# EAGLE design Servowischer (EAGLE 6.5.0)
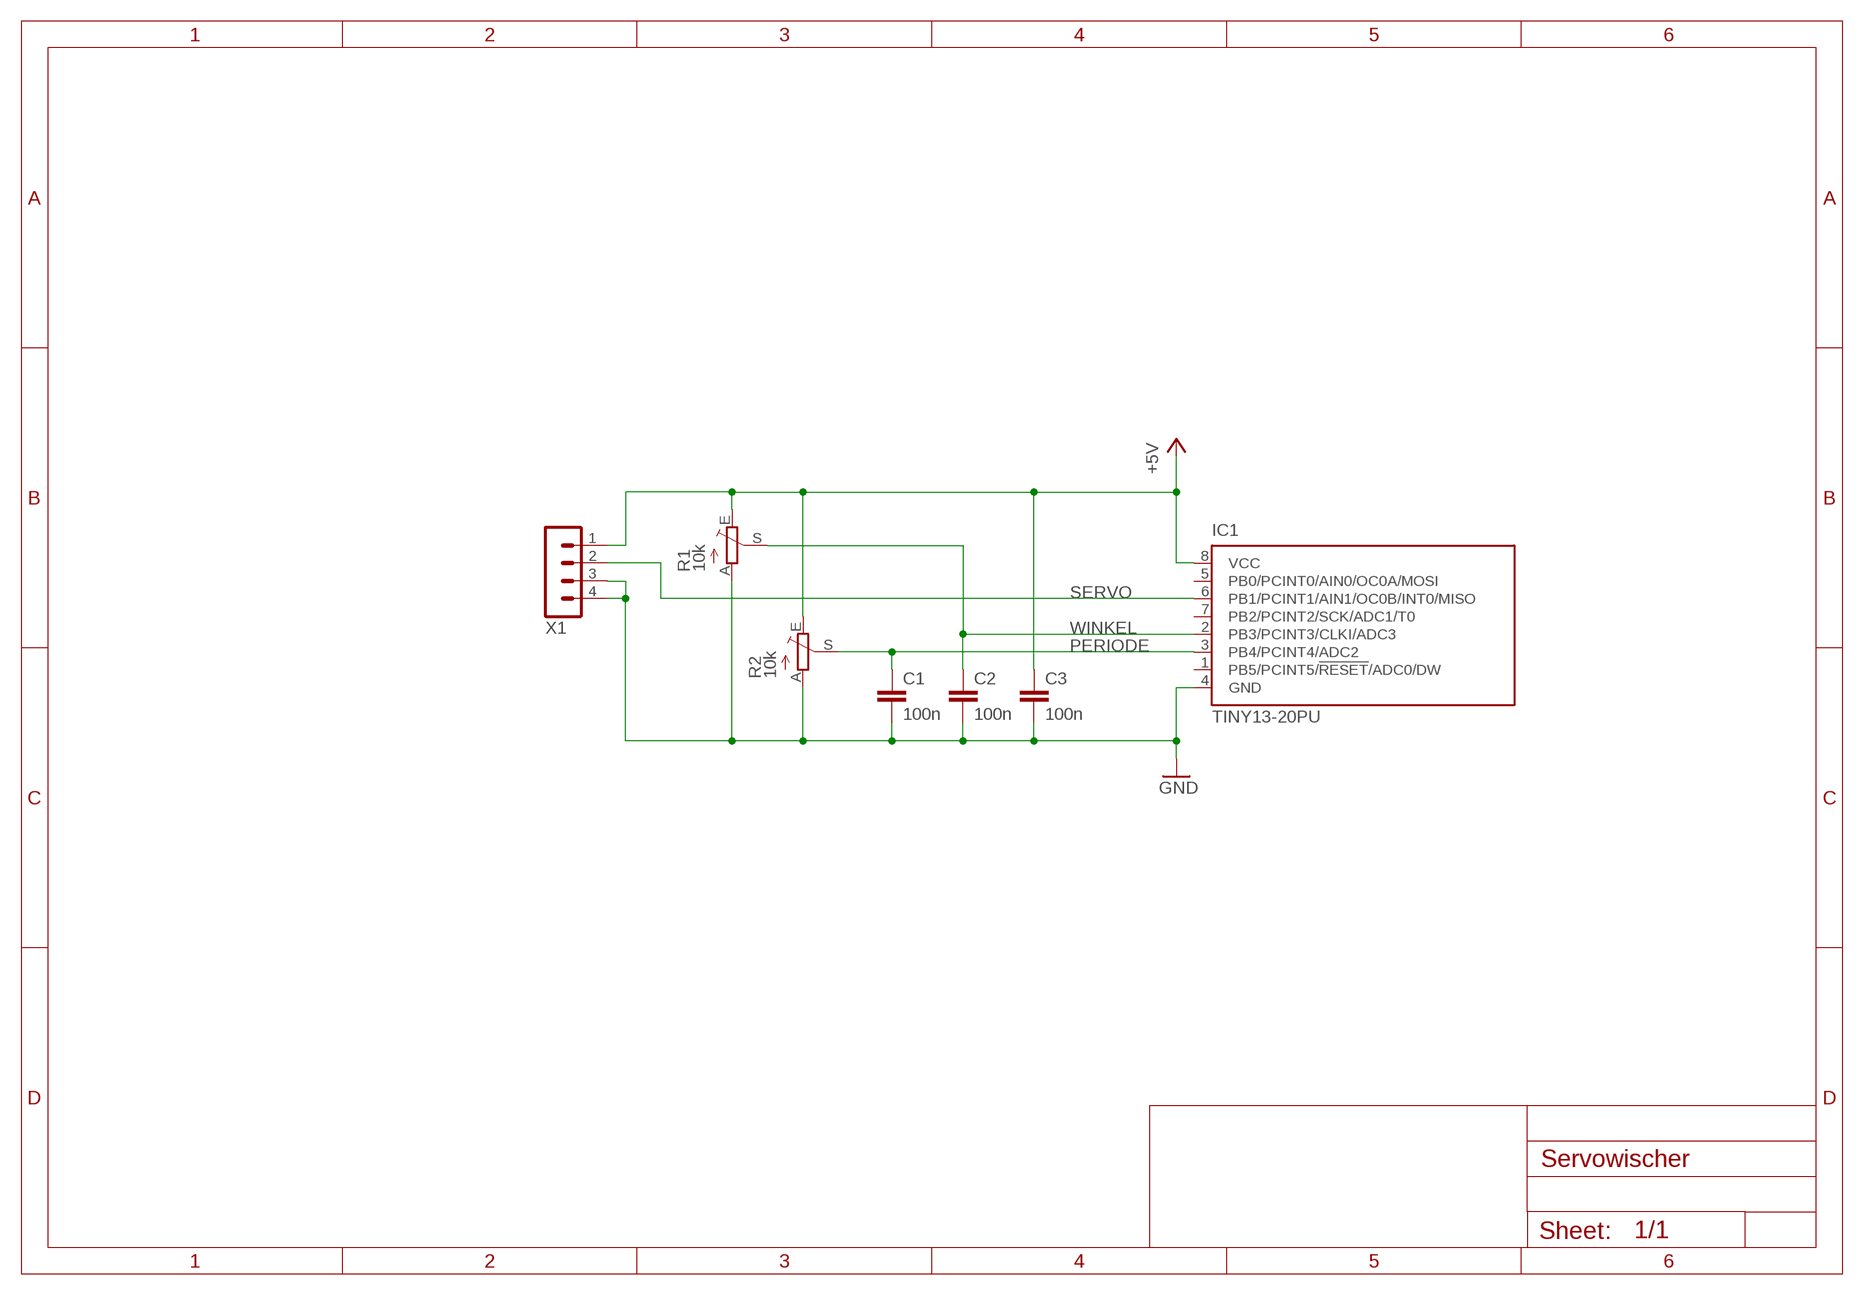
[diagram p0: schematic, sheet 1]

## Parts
C1  100n  C-EU050-024X044  [C050-024X044]
C2  100n  C-EU050-024X044  [C050-024X044]
C3  100n  C-EU050-024X044  [C050-024X044]
IC1  TINY13-20PU  [DIL08]
R1  10k  TRIM_EU-RJ9W  [RJ9W]
R2  10k  TRIM_EU-RJ9W  [RJ9W]
X1  MA04-1  [MA04-1]

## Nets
+5V: C3.1 IC1.8(VCC) R1.E R2.E X1.1
GND: C1.2 C2.2 C3.2 IC1.4(GND) R1.A R2.A X1.3 X1.4
PERIODE: C1.1 IC1.3(PB4/PCINT4/ADC2) R2.S
SERVO: IC1.6(PB1/PCINT1/AIN1/OC0B/INT0/MISO) X1.2
WINKEL: C2.1 IC1.2(PB3/PCINT3/CLKI/ADC3) R1.S
Unconnected: IC1.1(PB5/PCINT5/!RESET!/ADC0/DW) IC1.5(PB0/PCINT0/AIN0/OC0A/MOSI) IC1.7(PB2/PCINT2/SCK/ADC1/T0)

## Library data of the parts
C1-C3 = rcl:C-EU: CAPACITOR, European symbol
IC1 = atmel:TINY13: 8-bit AVR Microcontroller with 1K Bytes In-System Programmable Flash Source: http://www.atmel.com/dyn/resources/prod_documents/2535S.pdf; MPN: ATTINY13-20PU; OC_FARNELL: 9171550; OC_NEWARK: 96K6521
R1 R2 = pot:TRIM_EU-: POTENTIOMETER
X1 = con-lstb:MA04-1: PIN HEADER; OC_FARNELL: unknown; OC_NEWARK: unknown

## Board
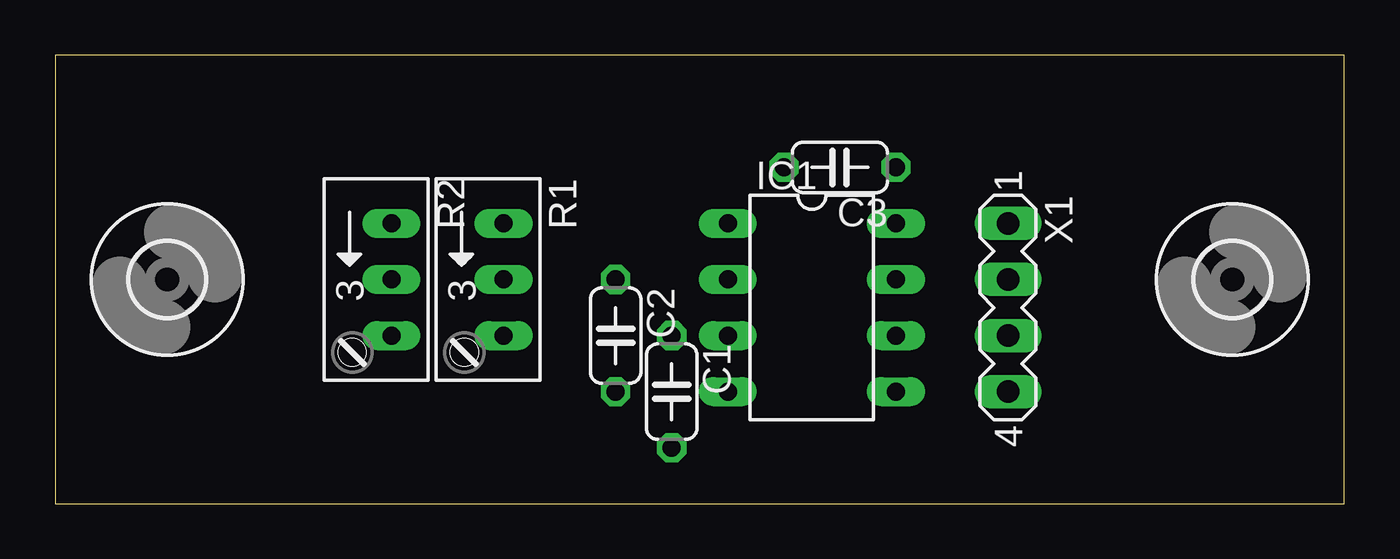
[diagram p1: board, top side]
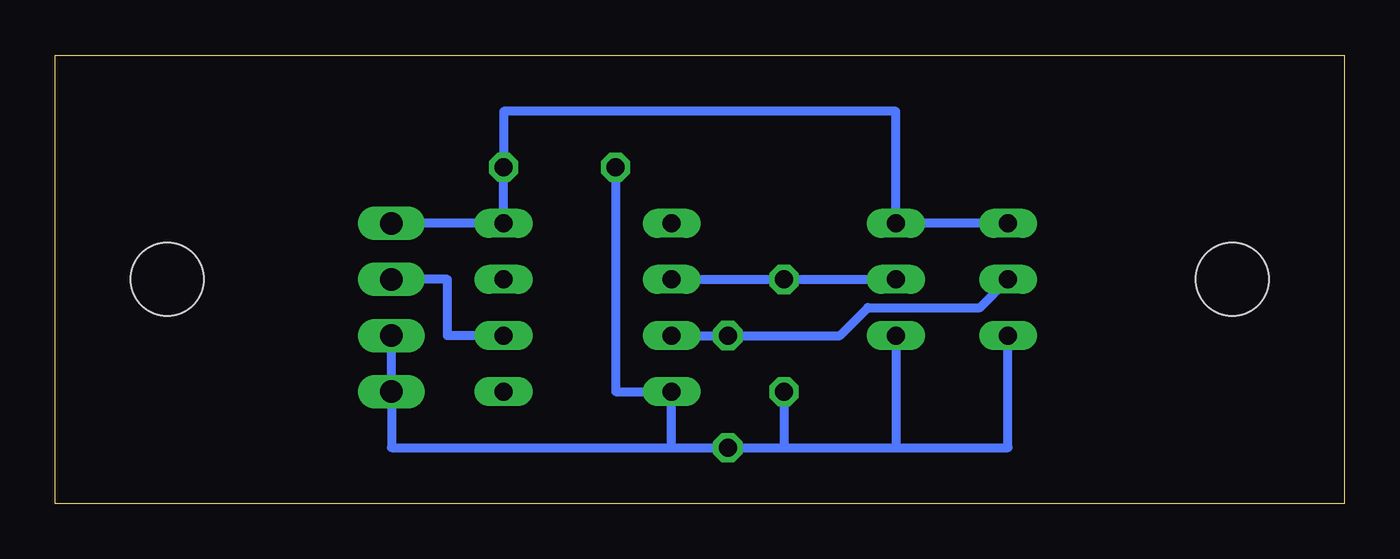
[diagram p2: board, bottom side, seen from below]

Size 58.42 x 20.32 mm. Coordinates in mm from the lower left corner, seen from the top.
Outline: 0,0 58.42,0 58.42,20.32 0,20.32 0,0
Copper layers (1*16): Top 0.035mm / dielectric 1.5mm / Bottom 0.035mm
Design rules "default": minimum track width 10mil, minimum drill 24mil, track to track 8mil, track to pad 8mil, pad to pad 8mil, via to via 8mil, smd to smd 8mil, copper to edge 40mil, drill to drill 8mil, minimum pad ring 10mil, minimum via ring 8mil, stop-mask expansion 4mil, vias tented up to drill 0mil, thermal gap 10mil

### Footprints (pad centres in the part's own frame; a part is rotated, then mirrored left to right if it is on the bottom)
C050-024X044 = drill 0.813 octagon: 1 -2.54,0; 2 2.54,0
DIL08 = drill 0.813 long: 1 -3.81,-3.81; 2 -1.27,-3.81; 3 1.27,-3.81; 4 3.81,-3.81; 5 3.81,3.81; 6 1.27,3.81; 7 -1.27,3.81; 8 -3.81,3.81
RJ9W = drill 0.813 long: A 2.54,0.635; E -2.54,0.635; S 0,0.635
3,3 = hole 3.3: 0,0
MA04-1 = drill 1.016 long: 1 -3.81,0; 2 -1.27,0; 3 1.27,0; 4 3.81,0

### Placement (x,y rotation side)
C1  27.94,5.08 270 top
C2  25.4,7.62 270 top
C3  35.56,15.24 180 top
IC1  34.29,8.89 270 top
R1  19.68,10.16 270 top
R2  14.61,10.16 270 top
U$1  [3,3]  5.08,10.16 0 top
U$2  [3,3]  53.34,10.16 0 top
X1  43.18,8.89 270 top

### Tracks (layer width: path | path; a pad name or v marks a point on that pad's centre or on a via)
+5V
  Bottom 0.406: X1.1 IC1.8 C3.1 38.1,17.78 20.32,17.78 R1.E R2.E
GND
  Bottom 0.406: X1.3 X1.4 43.18,2.54 30.48,2.54 | 30.48,2.54 IC1.4 33.02,5.08 C3.2 | 30.48,2.54 C1.2 25.4,2.54 | 25.4,2.54 20.32,2.54 | 20.32,2.54 15.24,2.54 R2.A | R1.A 20.32,2.54 | C2.2 25.4,2.54
PERIODE
  Bottom 0.406: IC1.3 C1.1 22.86,7.62 21.59,8.89 16.51,8.89 R2.S
SERVO
  Bottom 0.406: IC1.6 40.64,7.62 40.64,10.16 X1.2
WINKEL
  Bottom 0.406: IC1.2 C2.1 R1.S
